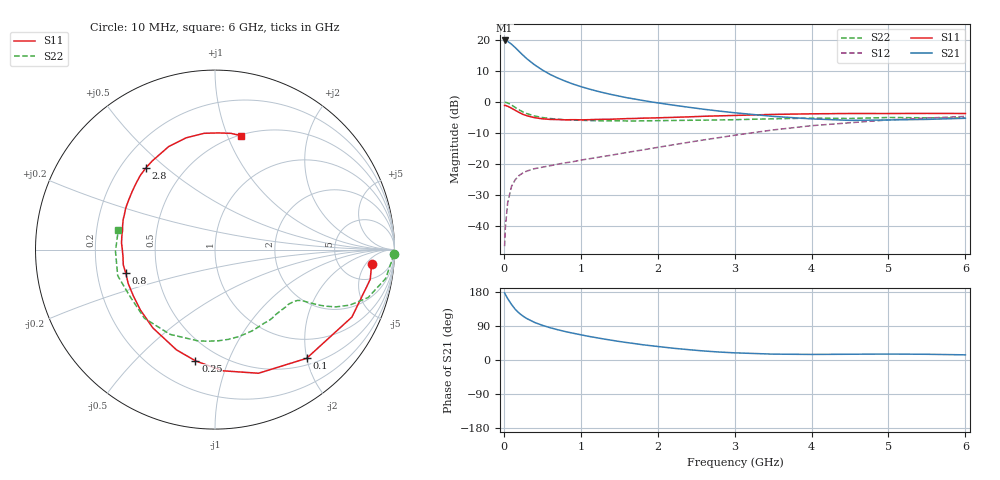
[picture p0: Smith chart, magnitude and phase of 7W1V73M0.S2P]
! Infineon Technologies  Discrete & RF Semiconductors
! BFS17W
! Si NPN RF Bipolar Junction Transistor in SOT323
! VCE = 1.75 V  IC = 3 mA
! Common Emitter S-Parameters:  August  1999
# GHz  S  MA  R  50
!  f  S11  S21  S12  S22
! GHz  MAG  ANG  MAG  ANG  MAG  ANG  MAG  ANG
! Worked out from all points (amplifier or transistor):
!   36 points, 10 MHz to 6 GHz, reference 50 ohm
!   highest |S21| = 19.9 dB at 10 MHz (marker M1)
!   |S21| within 3 dB of that: start of sweep to 176.6 MHz
!   unconditionally stable (mu >= 1): 672.6 MHz to end of sweep
!   at 250 MHz: K = 0.46, MSG = 19.0 dB, |S12| = -22.9 dB
!   at 1.4 GHz: K = 1.33, MAG = 6.3 dB, |S12| = -17.2 dB
!   at 6 GHz: K = 1.11, MAG = -2.3 dB, |S12| = -4.7 dB
!   S11 on the Smith chart (normalised r, x): 10 MHz: 10, -7; 100 MHz: 0.61, -2.00; 250 MHz: 0.37, -0.77; 800 MHz: 0.33, -0.12; 2.8 GHz: 0.30, +0.43; 6 GHz: 0.51, +1.12
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0.01  0.8766 -5.3  9.83 177.0  0.0047 83.6  0.9958 -1.5
0.02  0.8806 -10.9  9.778 172.8  0.0095 84.4  0.9854 -3.9
0.05  0.8504 -26.2  9.494 161.9  0.0236 76.4  0.9647 -9.6
0.1  0.7922 -49.9  8.544 146.5  0.0435 63.9  0.8938 -17.4
0.15  0.7303 -70.6  7.505 133.3  0.056 55.6  0.8121 -22.4
0.2  0.6764 -86.5  6.513 123.5  0.0653 50.5  0.7444 -25.4
0.25  0.629 -100.0  5.663 115.6  0.0717 45.7  0.6887 -27.2
0.3  0.5986 -111.0  4.974 109.2  0.0767 43.8  0.6488 -28.3
0.4  0.5571 -128.4  3.969 99.1  0.0838 41.3  0.5925 -29.6
0.5  0.5349 -140.9  3.282 91.6  0.0885 40.8  0.5608 -30.4
0.6  0.5228 -150.6  2.786 85.3  0.0933 41.9  0.5404 -31.6
0.8  0.5143 -165.2  2.163 75.0  0.1041 44.4  0.516 -35.3
0.9  0.518 -170.6  1.943 70.7  0.1086 45.7  0.5087 -37.2
1.1  0.5167 179.5  1.629 62.5  0.1205 48.5  0.5011 -42.0
1.3  0.5248 171.4  1.405 55.4  0.1325 51.1  0.4952 -47.5
1.6  0.5385 161.7  1.17 46.0  0.1528 54.1  0.4931 -56.0
2.2  0.5638 144.9  0.889 31.1  0.2033 58.4  0.5024 -74.9
2.8  0.5966 130.0  0.712 21.0  0.2658 58.3  0.5122 -94.8
3.5  0.6294 114.2  0.585 15.5  0.3532 54.2  0.5344 -117.9
4.5  0.6508 95.4  0.504 15.2  0.4612 42.5  0.5409 -151.4
5.5  0.6538 82.1  0.523 15.1  0.5492 30.8  0.5546 -179.0
6  0.6509 76.9  0.545 13.6  0.5837 25.1  0.5498 168.8
